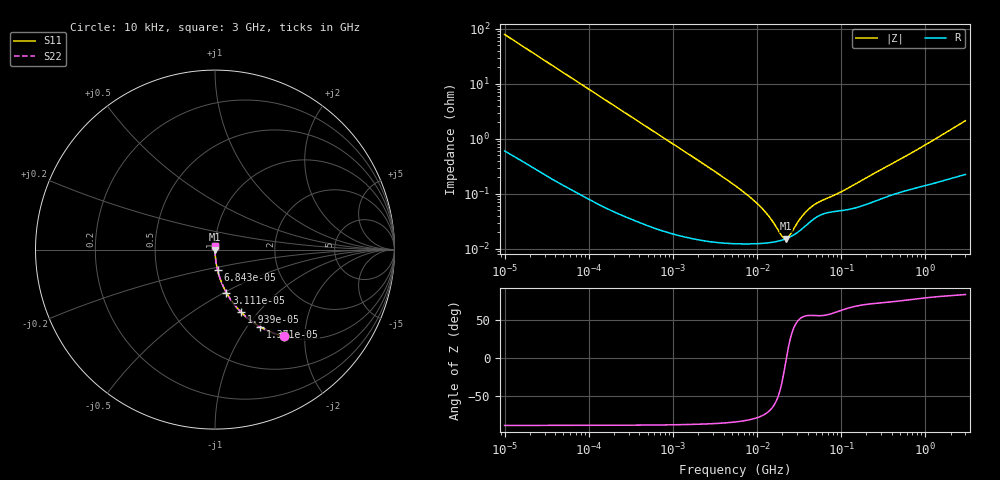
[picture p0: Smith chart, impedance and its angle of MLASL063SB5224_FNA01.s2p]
! MLASL063SB5224_FNA01  S-PARAMETER MODEL  ( Standard Model )
! Model Generated by TAIYO YUDEN Corporation (http://www.ty-top.com)
! Version 2.0
! TAIYO YUDEN Control No. 240306
! Copyright(c) 2009 TAIYO YUDEN CO.,LTD. All Rights Reserved.
! Product Description (link to TY-COMPAS)
! https://ds.yuden.co.jp/TYCOMPAS/or/detail?pn=MLASL063SB5224KFNA01&u=M
! Products Name : Multilayer Ceramic Capacitors
! Characteristics :
!  Capacitance : 0.22 [uF] , Rated Voltage : 10 [V] , TCC : X5R
!  Case Size : 0.6 x 0.3 / 0.024 x 0.012 [mm/inch] , Thickness : 0.3 / 0.012 [mm/inch]
!  (Conditions: Temperature = 25 [degC] , DC Bias Voltage = 0 [V])
! External Node Assignments :
!  1  o---| |---o  2
! GND o---------o GND
! Frequency Range : 10kHz  -  3GHz  [ 401 STEP ]
# MHZ S RI R 50
! Freq[MHz].  S11 Real  S11 Imag  S21 Real  S21 Imag  S12 Real  S12 Imag  S22 Real  S22 Imag
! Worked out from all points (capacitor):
!   401 points, 10 kHz to 3 GHz, reference 50 ohm
!   read as one part in series: C = 200 nF near 10.65 kHz
!   lowest |Z| = 15.2 mohm at 21.93 MHz (marker M1)
!   series resonance near 22.4 MHz, so ESL is about 250 pH
!   S11 on the Smith chart (normalised r, x): 10 kHz: 1.01, -1.59; 13.71 kHz: 1.01, -1.16; 19.39 kHz: 1.01, -0.82; 31.11 kHz: 1.00, -0.51; 68.43 kHz: 1.00, -0.23; 3 GHz: 1.00, +0.04
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0.01  0.387 -0.4833  0.613 0.4833  0.613 0.4833  0.387 -0.4833
0.013707  0.2531 -0.4309  0.7469 0.4309  0.7469 0.4309  0.2531 -0.4309
0.019389  0.1462 -0.3492  0.8538 0.3492  0.8538 0.3492  0.1462 -0.3492
0.031113  0.0634 -0.2396  0.9366 0.2396  0.9366 0.2396  0.0634 -0.2396
0.068432  0.0146 -0.1152  0.9854 0.1152  0.9854 0.1152  0.0146 -0.1152
0.082683  0.0102 -0.0959  0.9898 0.0959  0.9898 0.0959  0.0102 -0.0959
0.199902  0.00209 -0.0402  0.9979 0.0402  0.9979 0.0402  0.00209 -0.0402
0.683653  0.000363 -0.0119  0.9996 0.0119  0.9996 0.0119  0.000363 -0.0119
5.477226  0.000126 -0.00141  0.9999 0.00141  0.9999 0.00141  0.000126 -0.00141
8.252149  0.000124 -0.000862  0.9999 0.000862  0.9999 0.000862  0.000124 -0.000862
11.31085  0.000125 -0.000543  0.9999 0.000543  0.9999 0.000543  0.000125 -0.000543
14.55585  0.00013 -0.000328  0.9999 0.000328  0.9999 0.000328  0.00013 -0.000328
19.95104  0.000144 -8.6e-05  0.9999 8.6e-05  0.9999 8.6e-05  0.000144 -8.6e-05
21.93027  0.000151 -1.57e-05  0.9998 1.57e-05  0.9998 1.57e-05  0.000151 -1.57e-05
24.10585  0.000161 5.45e-05  0.9998 -5.45e-05  0.9998 -5.45e-05  0.000161 5.45e-05
31.02164  0.000204 0.000242  0.9998 -0.000242  0.9998 -0.000242  0.000204 0.000242
35.19136  0.000238 0.000333  0.9998 -0.000333  0.9998 -0.000333  0.000238 0.000333
45.28751  0.000331 0.000495  0.9997 -0.000495  0.9997 -0.000495  0.000331 0.000495
56.47134  0.00041 0.000605  0.9996 -0.000605  0.9996 -0.000605  0.00041 0.000605
109.4906  0.000504 0.00105  0.9995 -0.00105  0.9995 -0.00105  0.000504 0.00105
374.4521  0.000928 0.0032  0.9991 -0.0032  0.9991 -0.0032  0.000928 0.0032
3000  0.00269 0.0212  0.9973 -0.0212  0.9973 -0.0212  0.00269 0.0212
